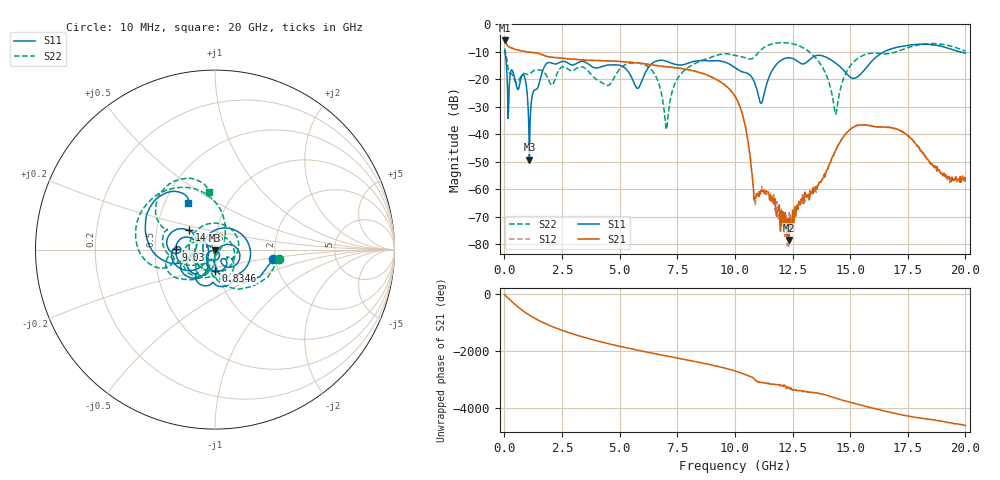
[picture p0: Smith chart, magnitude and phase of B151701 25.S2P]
!  2-Port S-parameters saved by WinCal
! VAR MeasName=S-Parameters (CALIBRATED_DATA) read from VNA (N5244A)
! VAR MeasDate=2015-12-24 19:11:04
! VAR NAME=B151701 25
! VAR FILENAME=B151701 25.S2P
! VAR DATE=2015-12-24 19:11:04
! VAR PHYS_PORTS=1,3
# Hz S DB R 50
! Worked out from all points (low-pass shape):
!   801 points, 10 MHz to 20 GHz, reference 50 ohm
!   highest |S21| = -5.92 dB at 10 MHz (marker M1); lowest = -78.4 dB at 12.35 GHz (marker M2)
!   |S21| within 3 dB of the highest: start of sweep to 393.5 MHz
!   lowest |S11| = -49.2 dB at 1.084 GHz (marker M3), VSWR 1.01, Z = 50 - j0.347 ohm
!   |S11| at or under -10 dB: 17.93 MHz to 16.47 GHz (16.46 GHz wide, 200 % of centre); 19.72 GHz to end of sweep
!   |S22| runs from -38.2 to -6.7 dB; largest |S21 - S12| = 0.0012
!   S11 on the Smith chart (normalised r, x): 10 MHz: 1.94, -0.24; 834.6 MHz: 0.98, -0.24; 9.03 GHz: 0.65, +0.00; 14.48 GHz: 0.73, +0.16; 20 GHz: 0.65, +0.37
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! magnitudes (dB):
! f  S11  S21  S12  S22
! 10 MHz  -9.7  -5.9  -5.9  -8.8
! 184.9 MHz  -29.9  -8.1  -8.1  -16.8
! 834.6 MHz  -18.4  -9.8  -9.8  -17.9
! 1.084 GHz  -49.2  -10.2  -10.2  -18.1
! 1.834 GHz  -14.3  -11.7  -11.7  -18.7
! 3.358 GHz  -13.5  -12.9  -12.9  -15.5
! 4.483 GHz  -14.9  -13.3  -13.3  -22.3
! 5.782 GHz  -23.3  -14.1  -14.1  -14.2
! 6.682 GHz  -13.2  -15.1  -15.1  -21.1
! 7.031 GHz  -13.5  -15.5  -15.5  -38.2
! 7.581 GHz  -14.8  -16.0  -16.0  -18.9
! 9.03 GHz  -13.3  -19.4  -19.4  -11.8
! 10.01 GHz  -15.8  -26.2  -26.2  -11.3
! 10.45 GHz  -17.6  -37.1  -37.1  -12.2
! 10.88 GHz  -21.8  -62.8  -65.8  -11.6
! 11.15 GHz  -28.7  -60.7  -60.6  -9.2
! 12.35 GHz  -12.2  -78.4  -68.5  -6.9
! 13.35 GHz  -12.1  -61.5  -61.6  -11.0
! 14.48 GHz  -14.8  -44.0  -44.0  -28.0
! 15.18 GHz  -19.6  -37.3  -37.3  -13.5
! 16.68 GHz  -9.2  -37.5  -37.5  -10.7
! 20 GHz  -10.5  -56.9  -57.0  -9.8
